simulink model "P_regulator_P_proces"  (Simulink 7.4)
settings: Solver=ode45  StartTime=0.0  StopTime=4  RelTol=1e-3

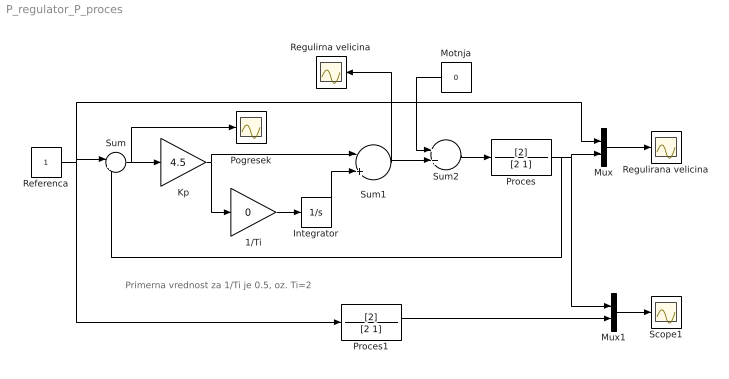
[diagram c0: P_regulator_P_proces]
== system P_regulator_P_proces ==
  note: Primerna vrednost za 1/Ti je 0.5, oz. Ti=2
  1/Ti : Gain  Gain=0  ParameterDataType=fixdt(1, 16)  ParameterScaling=2^0  OutDataType=fixdt(1, 16)  OutScaling=2^0
  Integrator : Integrator
  Kp : Gain  Gain=4.5  ParameterDataType=fixdt(1, 16)  ParameterScaling=2^0  OutDataType=fixdt(1, 16)  OutScaling=2^0
  Motnja : Constant  Value=0  OutDataType=fixdt(1, 16)  OutScaling=2^0
  Mux : Mux  Inputs=2
  Mux1 : Mux  Inputs=2
  Pogresek : Scope
  Proces : TransferFcn  Numerator=[2]  Denominator=[2 1]
  Proces1 : TransferFcn  Numerator=[2]  Denominator=[2 1]
  Referenca : Constant  OutDataType=fixdt(1, 16)  OutScaling=2^0
  Regulirana velicina : Scope
  Regulirna velicina : Scope
  Scope1 : Scope
  Sum : Sum  Inputs=|+-  OutDataType=fixdt(1, 16)  OutScaling=2^0
  Sum1 : Sum  Inputs=|++  OutDataType=fixdt(1, 16)  OutScaling=2^0
  Sum2 : Sum  OutDataType=fixdt(1, 16)  OutScaling=2^0
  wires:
  Referenca/1 -> Sum/1, Mux/1, Proces1/1
  Sum/1 -> Kp/1, Pogresek/1
  Proces/1 -> Sum/2, Mux/2, Mux1/1
  Mux/1 -> Regulirana velicina/1
  Proces1/1 -> Mux1/2
  Mux1/1 -> Scope1/1
  Kp/1 -> 1/Ti/1, Sum1/1
  1/Ti/1 -> Integrator/1
  Integrator/1 -> Sum1/2
  Sum1/1 -> Regulirna velicina/1, Sum2/2
  Sum2/1 -> Proces/1
  Motnja/1 -> Sum2/1
